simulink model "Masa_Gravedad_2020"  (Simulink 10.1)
settings: Solver=VariableStepAuto  StartTime=0.0  StopTime=10  MaxStep=0.001  RelTol=1e-3
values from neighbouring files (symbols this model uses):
  k = 50.0    (= 50)    [Modelo_MR_Gravedad.m]
  m = 2.0    (= 2)    [Modelo_MR_Gravedad.m]
  v0 = 0    [Modelo_MR_Gravedad.m]
  x0 = 0.5    [Modelo_MR_Gravedad.m]

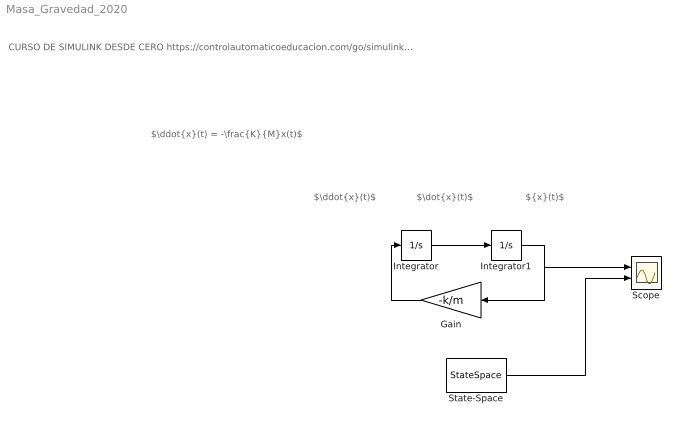
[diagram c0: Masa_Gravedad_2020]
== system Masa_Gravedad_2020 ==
  note: $\ddot{x}(t) = -\frac{K}{M}x(t)$
  note: CURSO DE SIMULINK DESDE CERO https://controlautomaticoeducacion.com/go/simulink-cupon/
  note: $\ddot{x}(t)$
  note: $\dot{x}(t)$
  note: ${x}(t)$
  Gain : Gain  Gain=-k/m
  Integrator : Integrator  InitialCondition=v0
  Integrator1 : Integrator  InitialCondition=x0
  Scope : Scope  NumInputPorts=2
  State-Space : StateSpace  A=[0, 1; -k/m, 0]  B=[0;0]  C=[1 0]  D=0  InitialCondition=[x0; v0]
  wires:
  Integrator/1 -> Integrator1/1
  Integrator1/1 -> Gain/1, Scope/1
  Gain/1 -> Integrator/1
  State-Space/1 -> Scope/2
